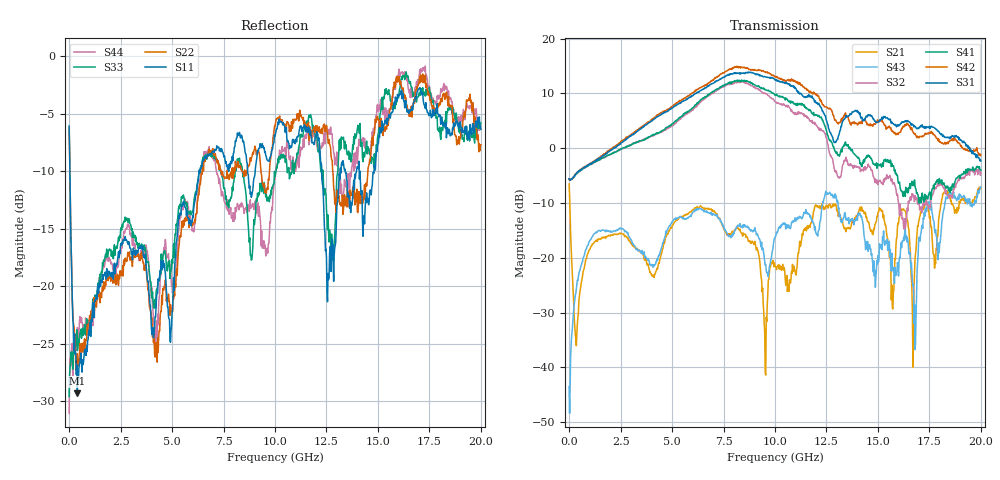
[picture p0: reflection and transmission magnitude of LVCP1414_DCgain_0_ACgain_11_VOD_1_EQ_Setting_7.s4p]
!Agilent Technologies,N5230A,MY46400459,A.07.50.48
!Agilent N5230A: A.07.50.48
!Date: Tuesday, April 17, 2012 18:31:55
!Correction: S11(Full 4 Port(1,2,3,4))
!S12(Full 4 Port(1,2,3,4))
!S13(Full 4 Port(1,2,3,4))
!S14(Full 4 Port(1,2,3,4))
!S21(Full 4 Port(1,2,3,4))
!S22(Full 4 Port(1,2,3,4))
!S23(Full 4 Port(1,2,3,4))
!S24(Full 4 Port(1,2,3,4))
!S31(Full 4 Port(1,2,3,4))
!S32(Full 4 Port(1,2,3,4))
!S33(Full 4 Port(1,2,3,4))
!S34(Full 4 Port(1,2,3,4))
!S41(Full 4 Port(1,2,3,4))
!S42(Full 4 Port(1,2,3,4))
!S43(Full 4 Port(1,2,3,4))
!S44(Full 4 Port(1,2,3,4))
!S4P File: Measurements: <S11,S12,S13,S14>,
!<S21,S22,S23,S24>,
!<S31,S32,S33,S34>,
!<S41,S42,S43,S44>:
# Hz S  dB  R 50
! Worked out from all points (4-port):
!   801 points, 300 kHz to 20 GHz, reference 50 ohm
!   strongest paths, dB at 300 kHz, 5 GHz, 10 GHz, 15 GHz, 20 GHz:
!     S31: -5.6, 7.3, 12.4, 4.8, -2.3
!     S42: -5.7, 7.7, 13.0, 5.1, -1.3
!     S41: -5.6, 4.5, 9.7, -2.9, -4.0
!     S32: -5.7, 4.1, 8.5, -6.7, -4.4
!     S43: -43.5, -13.4, -16.3, -19.6, -7.2
!     S21: -6.5, -14.2, -21.4, -11.7, -7.4
!   lowest |S11| = -29.3 dB at 400.3 MHz (marker M1), VSWR 1.07, Z = 53.2 + j1.54 ohm
!   |S11| at or under -10 dB: 37.74 MHz to 6.318 GHz (6.28 GHz wide, 198 % of centre); 12.26 GHz to 13.17 GHz (904.5 MHz wide, 7.11 % of centre); 14.13 GHz to 14.81 GHz (680.2 MHz wide, 4.7 % of centre)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
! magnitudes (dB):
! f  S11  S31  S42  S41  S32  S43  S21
! 300 kHz  -6.1  -5.6  -5.7  -5.6  -5.7  -43.5  -6.5
! 400.3 MHz  -29.3  -4.4  -4.4  -4.5  -4.5  -24.1  -32.0
! 10.08 GHz  -6.3  12.5  13.1  9.8  8.4  -15.3  -22.2
! 12.58 GHz  -18.9  4.2  7.3  2.2  0.7  -8.4  -10.9
! 16.8 GHz  -3.6  3.9  2.7  -6.8  -8.6  -36.8  -20.3
! 17.4 GHz  -4.9  3.8  2.7  -9.2  -9.9  -9.8  -10.2
! 20 GHz  -6.3  -2.3  -1.3  -4.0  -4.4  -7.2  -7.4
